ORGANIZATION_BLOCK "Blocco Organizzativo"
TITLE = "Main Program Sweep (Cycle)"
AUTHOR : MassimoZ
FAMILY : NovaSrl
VERSION : 0.1


VAR_TEMP
  OB1_EV_CLASS : BYTE ;	//Bits 0-3 = 1 (Coming event), Bits 4-7 = 1 (Event class 1)
  OB1_SCAN_1 : BYTE ;	//1 (Cold restart scan 1 of OB 1), 3 (Scan 2-n of OB 1)
  OB1_PRIORITY : BYTE ;	//1 (Priority of 1 is lowest)
  OB1_OB_NUMBR : BYTE ;	//1 (Organization block 1, OB1)
  OB1_RESERVED_1 : BYTE ;	//Reserved for system
  OB1_RESERVED_2 : BYTE ;	//Reserved for system
  OB1_PREV_CYCLE : INT ;	//Cycle time of previous OB1 scan (milliseconds)
  OB1_MIN_CYCLE : INT ;	//Minimum cycle time of OB1 (milliseconds)
  OB1_MAX_CYCLE : INT ;	//Maximum cycle time of OB1 (milliseconds)
  OB1_DATE_TIME : DATE_AND_TIME ;	//Date and time OB1 started
END_VAR
BEGIN
NETWORK
TITLE =Sempre 1

      UN    "ON";
      S     "ON";
NETWORK
TITLE =Gestione Posizioni Linea e Boxing

      UC    "Posizioni Linea";

NETWORK
TITLE =Gestione Consensi Linea e Boxing

      UC    "Consensi Linea";

NETWORK
TITLE =Gestione Contravers Zona Accatastatrice 1 piu' zona Bandiere

      O     "M25.0";

      O     "M25.1";
      O     "M25.2";
      CC    "Gest Contravers Acc.1 ZB";
NETWORK
TITLE =Gestione Contravers Zona Accatastatrice 2

      O     "M25.3";

      O     "M25.4";
      CC    "Gest Contravers Acc.2";
NETWORK
TITLE =Gestione Contravers Zona Accatastatrice 3

      O     "M25.6";
      O     "M25.7";
      CC    "Gest Contravers Acc.3";
NETWORK
TITLE =Gestione Contravers Zona apertura pallet

      U     "M25.5";

      CC    "Gest Contravers ZApertu";
NETWORK
TITLE =Gestione Pulsantiera pos carico 1 Acc. 1

      U     "M25.0";
      CC    "Puls. pos. carico1 Acc.1";
NETWORK
TITLE =Gestione Pulsantiera pos carico 2 Acc. 1

      U     "M25.1";
      CC    "Puls. pos. carico2 Acc.1";
NETWORK
TITLE =Gestione Pulsantiera pos carico 1 Acc. 2

      U     "M25.3";
      CC    "Puls. pos. carico1 Acc.2";
NETWORK
TITLE =Gestione Pulsantiera pos carico 2 Acc. 2

      U     "M25.4";
      CC    "Puls. pos. carico2 Acc.2";
NETWORK
TITLE =Gestione Pulsantiera pos carico 1 Acc. 3

      U     "M25.6";
      CC    "Puls. pos. carico1 Acc.3";
NETWORK
TITLE =Gestione Pulsantiera pos carico 2 Acc. 3

      U     "M25.7";
      CC    "Puls. pos.carico 2 Acc.3";
NETWORK
TITLE =Gestione Pulsantiera Zona Allineamento e Piega

      U     "M25.2";
      CC    "Puls. Allin. Piega Chius";
NETWORK
TITLE =Gestione Pulsantiera zona apertura pallet

      U     "M25.5";
      CC    "Puls. zona Apertura";
NETWORK
TITLE =Gestione Pulsantiera Boxing SX

      UN    "SL710";
      U(    ;
      O     "SL680";
      O     "M139.6";
      )     ;
      CC    "Pulsantiera Boxing SX";
NETWORK
TITLE =Gestione Pulsantiera Boxing DX

      UN    "SL710";
      U(    ;
      O     "PBoxingDX";
      O     "M139.6";
      )     ;
      CC    "Pulsantiera Boxing DX";
NETWORK
TITLE =Gestione Pulsantiera Robot Boxing Principale

      UN    "SL710";
      UN    "SL710B";
      CC    "Pulsantiera Robot Boxing";
NETWORK
TITLE =Gestione Automatico Linea

      UC    "Gest Automatico Linea";

NETWORK
TITLE =Gestione Automatico Boxing DX

      UC    "Gest Aut Boxing DX";

NETWORK
TITLE =Gestione Automatico Boxing SX

      UC    "Gest Aut Boxing SX";

NETWORK
TITLE =Gestione Automatico Robot Boxing DX

      U     "M201.1";
      U     "M206.1";
      U     "M211.1";
      U     "M216.1";
      CC    "Gest Aut Robot Boxing DX";
NETWORK
TITLE =Gestione Automatico Robot Boxing SX

      U     "M201.1";
      U     "M206.1";
      U     "M211.1";
      U     "M216.1";
      CC    "Gest Aut Robot Boxing SX";
NETWORK
TITLE =Gestione Avvisi ed Allarmi

      UC    "Gest Avvisi ed Allarmi";

NETWORK
TITLE =Gestione Interfacce con gli altri quadri

      UC    "Gest Interfacce";

NETWORK
TITLE =Gestione Reset linea

      UC    "Reset Linea";

NETWORK
TITLE =Gestione Output linea e Boxing

      U     DB90.DBX   21.0; // Da ricetta     DEP. FERMO COMPATTA PINZE= corto
      CC    "Output Linea e Boxing_2R";

      UN    DB90.DBX   21.0;
      CC    "Output Linea e Boxing_1R";

NETWORK
TITLE =Gestione Asse X Boxing

      UC    "Gest Asse X Boxing";

NETWORK
TITLE =Gestione Asse Y Boxing

      UC    "Gest Asse Y Boxing";

NETWORK
TITLE =Gestione Asse Z Boxing

      UC    "Gest Asse Z Boxing";

NETWORK
TITLE =Gestione Asse B Boxing

      UC    "Gest Asse B Boxing";

NETWORK
TITLE =

      UC    "FunzioniNonUsate";

NETWORK
TITLE =Gestione Scrittura Dati Asse X Boxing
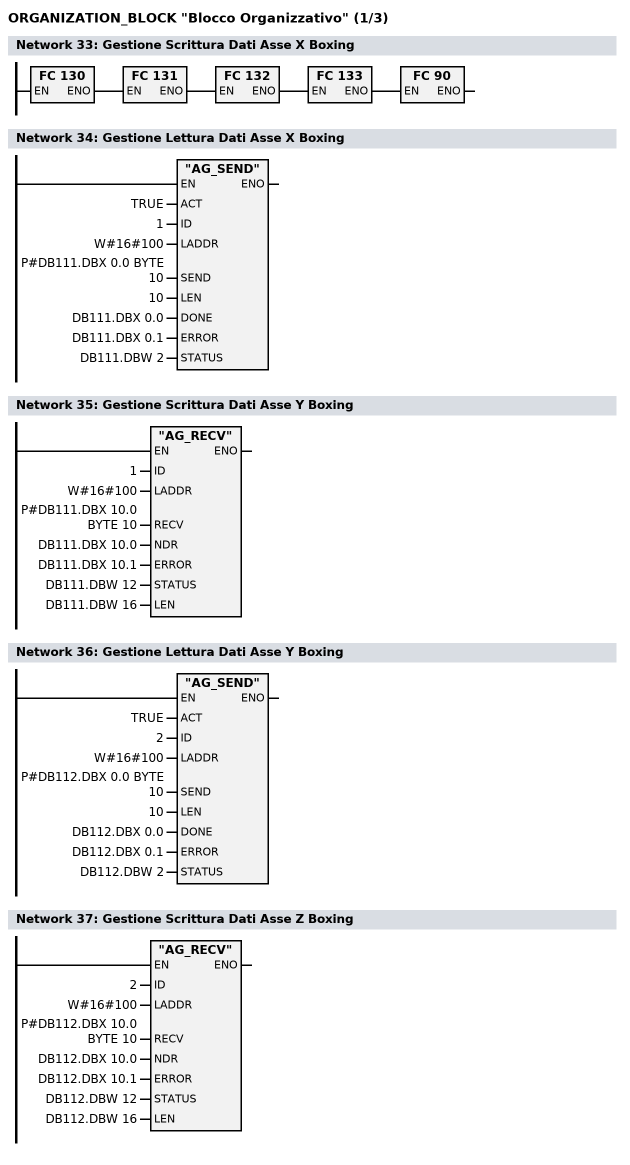
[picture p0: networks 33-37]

      CALL FC   130 ;
      CALL FC   131 ;
      CALL FC   132 ;
      CALL FC   133 ;
      CALL FC    90 ;
NETWORK
TITLE =Gestione Lettura Dati Asse X Boxing

      CALL "AG_SEND" (
           ACT                      := TRUE,
           ID                       := 1,
           LADDR                    := W#16#100,
           SEND                     := P#DB111.DBX 0.0 BYTE 10,
           LEN                      := 10,
           DONE                     := DB111.DBX    0.0,
           ERROR                    := DB111.DBX    0.1,
           STATUS                   := DB111.DBW    2);
NETWORK
TITLE =Gestione Scrittura Dati Asse Y Boxing

      CALL "AG_RECV" (
           ID                       := 1,
           LADDR                    := W#16#100,
           RECV                     := P#DB111.DBX 10.0 BYTE 10,
           NDR                      := DB111.DBX   10.0,
           ERROR                    := DB111.DBX   10.1,
           STATUS                   := DB111.DBW   12,
           LEN                      := DB111.DBW   16);
NETWORK
TITLE =Gestione Lettura Dati Asse Y Boxing

      CALL "AG_SEND" (
           ACT                      := TRUE,
           ID                       := 2,
           LADDR                    := W#16#100,
           SEND                     := P#DB112.DBX 0.0 BYTE 10,
           LEN                      := 10,
           DONE                     := DB112.DBX    0.0,
           ERROR                    := DB112.DBX    0.1,
           STATUS                   := DB112.DBW    2);
NETWORK
TITLE =Gestione Scrittura Dati Asse Z Boxing

      CALL "AG_RECV" (
           ID                       := 2,
           LADDR                    := W#16#100,
           RECV                     := P#DB112.DBX 10.0 BYTE 10,
           NDR                      := DB112.DBX   10.0,
           ERROR                    := DB112.DBX   10.1,
           STATUS                   := DB112.DBW   12,
           LEN                      := DB112.DBW   16);
NETWORK
TITLE =Gestione Lettura Dati Asse Z Boxing
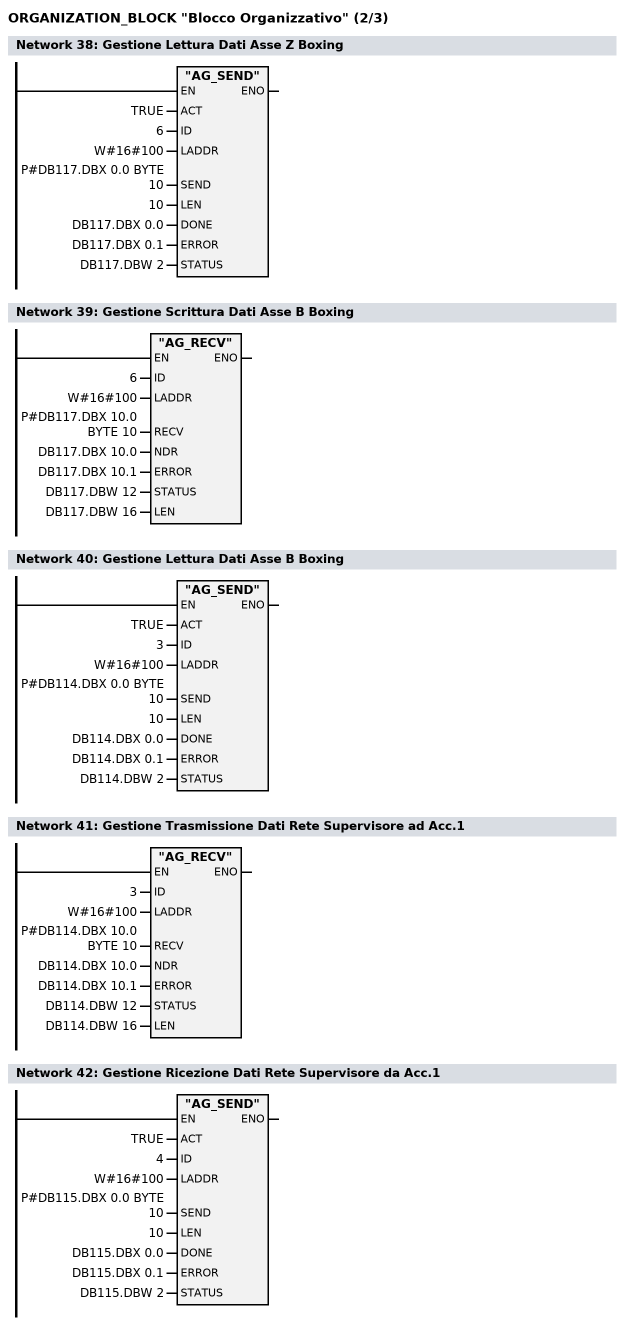
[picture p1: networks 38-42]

      CALL "AG_SEND" (
           ACT                      := TRUE,
           ID                       := 6,
           LADDR                    := W#16#100,
           SEND                     := P#DB117.DBX 0.0 BYTE 10,
           LEN                      := 10,
           DONE                     := DB117.DBX    0.0,
           ERROR                    := DB117.DBX    0.1,
           STATUS                   := DB117.DBW    2);
NETWORK
TITLE =Gestione Scrittura Dati Asse B Boxing

      CALL "AG_RECV" (
           ID                       := 6,
           LADDR                    := W#16#100,
           RECV                     := P#DB117.DBX 10.0 BYTE 10,
           NDR                      := DB117.DBX   10.0,
           ERROR                    := DB117.DBX   10.1,
           STATUS                   := DB117.DBW   12,
           LEN                      := DB117.DBW   16);
NETWORK
TITLE =Gestione Lettura Dati Asse B Boxing

      CALL "AG_SEND" (
           ACT                      := TRUE,
           ID                       := 3,
           LADDR                    := W#16#100,
           SEND                     := P#DB114.DBX 0.0 BYTE 10,
           LEN                      := 10,
           DONE                     := DB114.DBX    0.0,
           ERROR                    := DB114.DBX    0.1,
           STATUS                   := DB114.DBW    2);
NETWORK
TITLE =Gestione Trasmissione Dati Rete Supervisore ad Acc.1

      CALL "AG_RECV" (
           ID                       := 3,
           LADDR                    := W#16#100,
           RECV                     := P#DB114.DBX 10.0 BYTE 10,
           NDR                      := DB114.DBX   10.0,
           ERROR                    := DB114.DBX   10.1,
           STATUS                   := DB114.DBW   12,
           LEN                      := DB114.DBW   16);
NETWORK
TITLE =Gestione Ricezione Dati Rete Supervisore da Acc.1

      CALL "AG_SEND" (
           ACT                      := TRUE,
           ID                       := 4,
           LADDR                    := W#16#100,
           SEND                     := P#DB115.DBX 0.0 BYTE 10,
           LEN                      := 10,
           DONE                     := DB115.DBX    0.0,
           ERROR                    := DB115.DBX    0.1,
           STATUS                   := DB115.DBW    2);

NETWORK
TITLE =Gestione Trasmissione Dati Rete Supervisore ad Acc.2
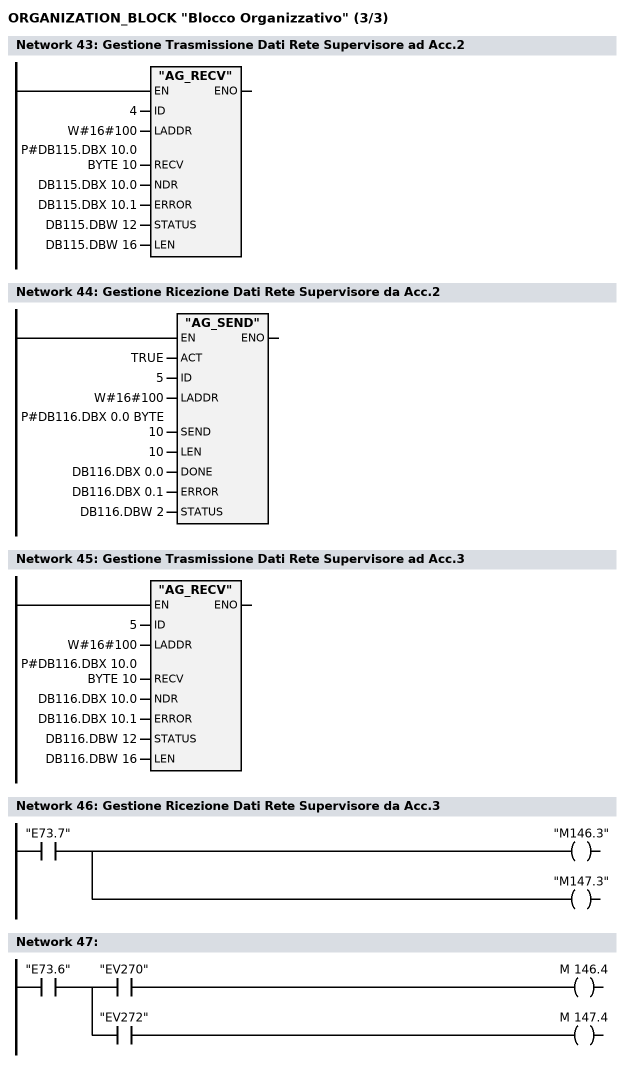
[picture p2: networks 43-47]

      CALL "AG_RECV" (
           ID                       := 4,
           LADDR                    := W#16#100,
           RECV                     := P#DB115.DBX 10.0 BYTE 10,
           NDR                      := DB115.DBX   10.0,
           ERROR                    := DB115.DBX   10.1,
           STATUS                   := DB115.DBW   12,
           LEN                      := DB115.DBW   16);
NETWORK
TITLE =Gestione Ricezione Dati Rete Supervisore da Acc.2

      CALL "AG_SEND" (
           ACT                      := TRUE,
           ID                       := 5,
           LADDR                    := W#16#100,
           SEND                     := P#DB116.DBX 0.0 BYTE 10,
           LEN                      := 10,
           DONE                     := DB116.DBX    0.0,
           ERROR                    := DB116.DBX    0.1,
           STATUS                   := DB116.DBW    2);

NETWORK
TITLE =Gestione Trasmissione Dati Rete Supervisore ad Acc.3

      CALL "AG_RECV" (
           ID                       := 5,
           LADDR                    := W#16#100,
           RECV                     := P#DB116.DBX 10.0 BYTE 10,
           NDR                      := DB116.DBX   10.0,
           ERROR                    := DB116.DBX   10.1,
           STATUS                   := DB116.DBW   12,
           LEN                      := DB116.DBW   16);
NETWORK
TITLE =Gestione Ricezione Dati Rete Supervisore da Acc.3

      U     "E73.7";
      =     "M146.3";
      =     "M147.3";
NETWORK
TITLE =


      U     "E73.6";
      =     L     20.0;
      U     L     20.0;
      U     "EV270";
      =     M    146.4;
      U     L     20.0;
      U     "EV272";
      =     M    147.4;
NETWORK
TITLE =
//Remmato la condizione per il SPBN A92.6

// U     "A92.6"
      SPBN  M001;
      L     1;
      T     DB3.DBW    0;
      SPA   M002;
M001: L     0;
      T     DB3.DBW    0;
M002: NOP   0;
NETWORK
TITLE =Gestione Trasmissione Dati Rete Supervisore ad Foratrice
//Remmato la condizione per il SPBN A92.7
//  U     "A92.7"
      SPBN  M003;
      L     2;
      T     DB3.DBW    2;
      SPA   M004;
M003: L     0;
      T     DB3.DBW    2;
M004: NOP   0;
NETWORK
TITLE =Abilita modifiche per rotazione pinza 2

      U     "ON";
      =     "ENAB_ROT_2";
END_ORGANIZATION_BLOCK

